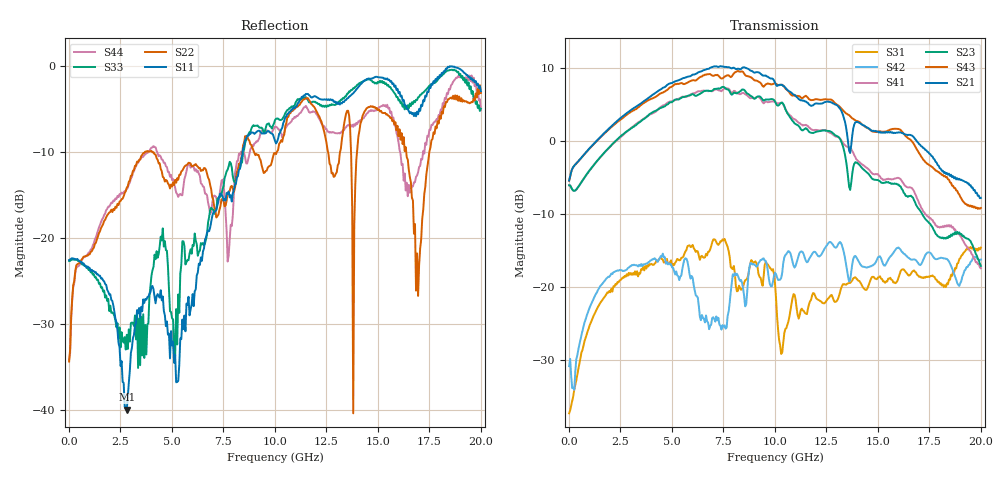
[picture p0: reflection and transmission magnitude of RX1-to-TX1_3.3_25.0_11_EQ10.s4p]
!Agilent Technologies,N5225A,MY51451112,A.09.50.13
!Agilent N5225A: A.09.50.13
!Date: Wednesday, January 31, 2018 11:05:00
!Correction: S11(Full 4 Port(1,2,3,4))
!S12(Full 4 Port(1,2,3,4))
!S13(Full 4 Port(1,2,3,4))
!S14(Full 4 Port(1,2,3,4))
!S21(Full 4 Port(1,2,3,4))
!S22(Full 4 Port(1,2,3,4))
!S23(Full 4 Port(1,2,3,4))
!S24(Full 4 Port(1,2,3,4))
!S31(Full 4 Port(1,2,3,4))
!S32(Full 4 Port(1,2,3,4))
!S33(Full 4 Port(1,2,3,4))
!S34(Full 4 Port(1,2,3,4))
!S41(Full 4 Port(1,2,3,4))
!S42(Full 4 Port(1,2,3,4))
!S43(Full 4 Port(1,2,3,4))
!S44(Full 4 Port(1,2,3,4))
!S4P File: Measurements: <S11,S12,S13,S14>,
!<S21,S22,S23,S24>,
!<S31,S32,S33,S34>,
!<S41,S42,S43,S44>:
# Hz S  RI  R 50
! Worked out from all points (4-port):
!   401 points, 10 MHz to 20 GHz, reference 50 ohm
!   strongest paths, dB at 10 MHz, 5.008 GHz, 10.01 GHz, 15 GHz, 20 GHz:
!     S21: -5.4, 7.9, 8.0, 1.3, -7.8
!     S43: -5.5, 7.4, 7.9, 1.3, -9.2
!     S23: -6.1, 5.3, 5.4, -5.3, -17.1
!     S41: -6.1, 5.4, 5.3, -4.5, -17.4
!     S42: -30.8, -17.3, -18.0, -15.9, -16.2
!     S31: -37.2, -17.2, -19.4, -18.7, -14.6
!   lowest |S11| = -40.0 dB at 2.809 GHz (marker M1), VSWR 1.02, Z = 49.7 - j0.953 ohm
!   |S11| at or under -10 dB: start of sweep to 8.433 GHz
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1e7  -0.0742 -0.00296  -0.000152 0.0006  0.0135 0.000746  -0.000147 0.000601
     0.5363 0.0119  -0.013 0.0139  -0.4978 -0.000396  0.0266 0.0122
     0.0138 0.00069  -0.000176 0.000696  -0.0732 -0.00401  -0.00025 0.000201
     -0.4977 0.000699  0.0263 0.0121  0.5338 0.0108  -0.0132 0.0145
2.8086e9  -0.00282 -0.00959  0.0166 0.00261  0.0545 0.1099  0.018 0.000222
          1.228 -0.9415  0.1961 0.00288  -0.8732 0.7673  0.1033 0.0917
          0.0601 0.1071  0.0198 0.00325  0.0146 0.0231  0.0215 0.000515
          -0.7545 0.8765  0.0906 0.0958  0.9699 -1.16  0.1867 -0.0494
7.0065e9  -0.0312 0.1365  0.0142 -0.0155  0.1351 0.067  0.0088 -0.0303
          -3.203 0.2144  0.1071 -0.1278  2.173 -0.5064  0.0375 0.0285
          0.1643 0.134  0.0233 -0.0158  0.0228 0.1445  0.0221 -0.0358
          1.762 -1.325  0.0617 -0.00973  -2.334 1.512  0.0932 -0.1459
8.655675e9  -0.00263 0.3921  0.00351 -0.00846  0.0763 0.0675  -0.0076 -0.0173
            -0.789 3.017  -0.1156 0.3759  0.1471 -2.102  -0.00581 0.1324
            0.0955 0.0641  0.0092 -0.0203  0.0337 0.3925  -0.0117 -0.0291
            -0.811 -1.874  -0.0305 0.0879  0.8176 2.65  0.1964 0.1872
1.050475e10  0.1569 0.4795  -0.0287 -0.0334  0.0099 0.0184  -0.0488 -0.00311
             1.975 1.203  0.3035 0.3297  -1.592 -0.438  0.0528 0.1901
             -0.0234 0.0463  -0.0363 -0.0305  0.2258 0.4833  -0.0539 -0.00886
             -1.6 0.4378  0.0824 0.144  2.278 -0.1366  0.4183 -0.1072
1.42029e10  0.6697 0.4216  -0.0285 0.000259  0.00581 0.0932  -0.0123 0.0127
            0.2646 -1.273  0.4569 0.1507  0.0683 0.6561  0.1504 0.0355
            0.0167 0.1031  -0.0134 -0.0016  0.7625 0.268  -0.023 0.0173
            0.5875 0.3754  0.1284 0.0562  -1.04 -0.7912  -0.1516 -0.4611
2e10  0.7117 0.0697  0.023 0.0349  -0.0796 0.1607  0.0349 0.0208
      0.0232 0.4072  0.6935 0.0749  0.00767 -0.1396  0.1541 0.0403
      -0.079 0.1691  0.00638 0.0478  0.564 -0.025  0.0476 0.0206
      -0.1262 -0.0476  0.1478 0.0458  0.3311 0.1083  -0.1519 -0.5316
